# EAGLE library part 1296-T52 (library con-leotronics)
1.27mm SINGLE ROW FEMALE SOCKET Source: http://www.leotronics.co.uk/Conexcon/Data%20Sheets/sec.%20A/1296ing.pdf
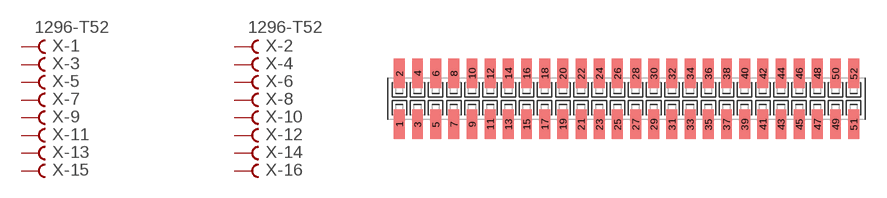
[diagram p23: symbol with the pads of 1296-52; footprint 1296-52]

Designator prefix X; gates -1=FVAL -2=FVAL -3=F -4=F -5=F -6=F -7=F -8=F -9=F -10=F -11=F -12=F -13=F -14=F -15=F -16=F -17=F -18=F -19=F -20=F -21=F -22=F -23=F -24=F -25=F -26=F -27=F -28=F -29=F -30=F -31=F -32=F -33=F -34=F -35=F -36=F -37=F -38=F -39=F -40=F -41=F -42=F -43=F -44=F -45=F -46=F -47=F -48=F -49=F -50=F -51=F -52=F

## 1296-T52 (OC_FARNELL: unknown; OC_NEWARK: unknown)  [1296-52]
1  -1:B  pas
2  -2:B  pas
3  -3:B  pas
4  -4:B  pas
5  -5:B  pas
6  -6:B  pas
7  -7:B  pas
8  -8:B  pas
9  -9:B  pas
10  -10:B  pas
11  -11:B  pas
12  -12:B  pas
13  -13:B  pas
14  -14:B  pas
15  -15:B  pas
16  -16:B  pas
17  -17:B  pas
18  -18:B  pas
19  -19:B  pas
20  -20:B  pas
21  -21:B  pas
22  -22:B  pas
23  -23:B  pas
24  -24:B  pas
25  -25:B  pas
26  -26:B  pas
27  -27:B  pas
28  -28:B  pas
29  -29:B  pas
30  -30:B  pas
31  -31:B  pas
32  -32:B  pas
33  -33:B  pas
34  -34:B  pas
35  -35:B  pas
36  -36:B  pas
37  -37:B  pas
38  -38:B  pas
39  -39:B  pas
40  -40:B  pas
41  -41:B  pas
42  -42:B  pas
43  -43:B  pas
44  -44:B  pas
45  -45:B  pas
46  -46:B  pas
47  -47:B  pas
48  -48:B  pas
49  -49:B  pas
50  -50:B  pas
51  -51:B  pas
52  -52:B  pas

## Footprint 1296-52 (pad centres in mm)
1.27mm SINGLE ROW FEMALE SOCKET Source: http://www.leotronics.co.uk/Conexcon/Data%20Sheets/sec.%20A/1296ing.pdf
smd 0.76 x 2.05: 1 -15.875,-1.78; 2 -15.875,1.78; 3 -14.605,-1.78; 4 -14.605,1.78; 5 -13.335,-1.78; 6 -13.335,1.78; 7 -12.065,-1.78; 8 -12.065,1.78; 9 -10.795,-1.78; 10 -10.795,1.78; 11 -9.525,-1.78; 12 -9.525,1.78; 13 -8.255,-1.78; 14 -8.255,1.78; 15 -6.985,-1.78; 16 -6.985,1.78; 17 -5.715,-1.78; 18 -5.715,1.78; 19 -4.445,-1.78; 20 -4.445,1.78; 21 -3.175,-1.78; 22 -3.175,1.78; 23 -1.905,-1.78; 24 -1.905,1.78; 25 -0.635,-1.78; 26 -0.635,1.78; 27 0.635,-1.78; 28 0.635,1.78; 29 1.905,-1.78; 30 1.905,1.78; 31 3.175,-1.78; 32 3.175,1.78; 33 4.445,-1.78; 34 4.445,1.78; 35 5.715,-1.78; 36 5.715,1.78; 37 6.985,-1.78; 38 6.985,1.78; 39 8.255,-1.78; 40 8.255,1.78; 41 9.525,-1.78; 42 9.525,1.78; 43 10.795,-1.78; 44 10.795,1.78; 45 12.065,-1.78; 46 12.065,1.78; 47 13.335,-1.78; 48 13.335,1.78; 49 14.605,-1.78; 50 14.605,1.78; 51 15.875,-1.78; 52 15.875,1.78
